(* Logix 5000 Rung export; software revision 16.03 *)

MODULES
   Local : vendor None type None code None
   MCMAOI : vendor None type None code None
END_MODULES

TYPE MCMSTATUS :
STRUCT
   PassCnt : INT;
   Product : INT[2];
   Rev : INT[2];
   OP : INT[2];
   Run : INT[2];
   Prt1Errs : MCMPortErrors;
   Prt2Errs : MCMPortErrors;
   Blk : MCMBlkStat;
   Port1LastErr : INT;
   Port1PreviousErr : INT;
   Port2LastErr : INT;
   Port2PreviousErr : INT;
END_STRUCT
END_TYPE

TYPE MCMCONFIG :
STRUCT
   ModDef : MCMModule;
   Port1 : MCMPort;
   Port2 : MCMPort;
   Port1MasterCmd : MCMCmd[100];
   Port2MasterCmd : MCMCmd[100];
END_STRUCT
END_TYPE

TYPE _CoilArray :
STRUCT
   Boolean : BOOL[416];
END_STRUCT
END_TYPE

TYPE MCMPortErrors :
STRUCT
   CmdReq : INT;
   CmdResp : INT;
   CmdErr : INT;
   Requests : INT;
   Responses : INT;
   ErrSent : INT;
   ErrRec : INT;
END_STRUCT
END_TYPE

TYPE _CmdControl :
STRUCT
   TriggerCmdCntrl : BOOL;
   NumberOfCommands : INT;
   PortNumber : INT;
   CommandIndex : INT[6];
   CmdsAddedToQueue : INT;
   CmdControlBlockID : INT;
   CmdCntrlPending : BOOL;
END_STRUCT
END_TYPE

TYPE _EventCmd :
STRUCT
   EventCmdTrigger : BOOL;
   EventCmdPending : BOOL;
   PortNumber : INT;
   SlaveAddress : INT;
   InternalDBAddress : INT;
   PointCount : INT;
   SwapCode : INT;
   ModbusFunctionCode : INT;
   DeviceDBAddress : INT;
   EventCmdStatusReturned : INT;
   EventBlockID : INT;
END_STRUCT
END_TYPE

TYPE _SlavePollStatus :
STRUCT
   Port1Slave0Read : BOOL;
   Port1Slave128Read : BOOL;
   Port2Slave0Read : BOOL;
   Port2Slave128Read : BOOL;
   P1Slaves : INT[256];
   P2Slaves : INT[256];
END_STRUCT
END_TYPE

TYPE MCMPort :
STRUCT
   Enabled : INT;
   Type : INT;
   FloatFlag : INT;
   FloatStart : INT;
   FloatOffset : INT;
   Protocol : INT;
   Baudrate : INT;
   Parity : INT;
   DataBits : INT;
   StopBits : INT;
   RTSOn : INT;
   RTSOff : INT;
   MinResp : INT;
   UseCTS : INT;
   SlaveID : INT;
   BitInOffset : INT;
   WordInOffset : INT;
   OutOffset : INT;
   HoldOffset : INT;
   CmdCount : INT;
   MinCmdDelay : INT;
   CmdErrPtr : INT;
   RespTO : INT;
   RetryCount : INT;
   ErrorDelayCntr : INT;
   Reserved : INT;
   InterCharacterDelay : INT;
   Fcn99Offset : INT;
END_STRUCT
END_TYPE

TYPE MCMModuleDef :
STRUCT
   CONFIG : MCMCONFIG;
   DATA : MCMDATA;
   STATUS : MCMSTATUS;
   CONTROL : MCMCONTROL;
   _UTIL : _Util;
END_STRUCT
END_TYPE

TYPE MCMCONTROL :
STRUCT
   WarmBoot : BOOL;
   ColdBoot : BOOL;
   BPLastRead : INT;
   BPLastWrite : INT;
   BlockIndex : INT;
   ReadDataSize : DINT;
   MaxReadBlock : DINT;
   WriteDataSize : DINT;
   MaxWriteBlock : DINT;
END_STRUCT
END_TYPE

TYPE MCMModule :
STRUCT
   WriteStartReg : INT;
   WriteRegCnt : INT;
   ReadStartReg : INT;
   ReadRegCnt : INT;
   BPFail : INT;
   ErrStatPtr : INT;
END_STRUCT
END_TYPE

TYPE _Passthru :
STRUCT
   MBOffset : INT;
   MBOffsetBit : INT;
   MBMsgLen : INT;
   MBMsg : SINT[500];
   MBControl1 : CONTROL;
   MBControl2 : CONTROL;
   MBScratch : INT[3];
   MBCoil : _CoilArray;
END_STRUCT
END_TYPE

TYPE MCMDATA :
STRUCT
   ReadData : INT[600];
   WriteData : INT[600];
END_STRUCT
END_TYPE

TYPE MCMBlkStat :
STRUCT
   Read : INT;
   Write : INT;
   Parse : INT;
   Event : INT;
   Cmd : INT;
   Err : INT;
END_STRUCT
END_TYPE

TYPE MCMCmd :
STRUCT
   Enable : INT;
   IntAddress : INT;
   PollInt : INT;
   Count : INT;
   Swap : INT;
   Node : INT;
   Func : INT;
   DevAddress : INT;
END_STRUCT
END_TYPE

TYPE _Util :
STRUCT
   CmdControl : _CmdControl;
   EventCmd : _EventCmd;
   SlavePollStat : _SlavePollStatus;
   Passthru : _Passthru;
END_STRUCT
END_TYPE

ADD_ON_INSTRUCTION PSMCM   (* revision 2.2, vendor ProSoft Technology Inc., ExecutePrescan *)
// Revision note:
// Added viewing capability for the Add_On Instruction
VAR_IN_OUT
   Local_C : SINT[400]; {required}
   Local_Input : INT[250]; {required}
   Local_Output : INT[248]; {required}
   MCM : MCMModuleDef; {required}
END_VAR
VAR
   MJFAULTS : DINT[12];
END_VAR

ROUTINE Logic   (* ladder *)
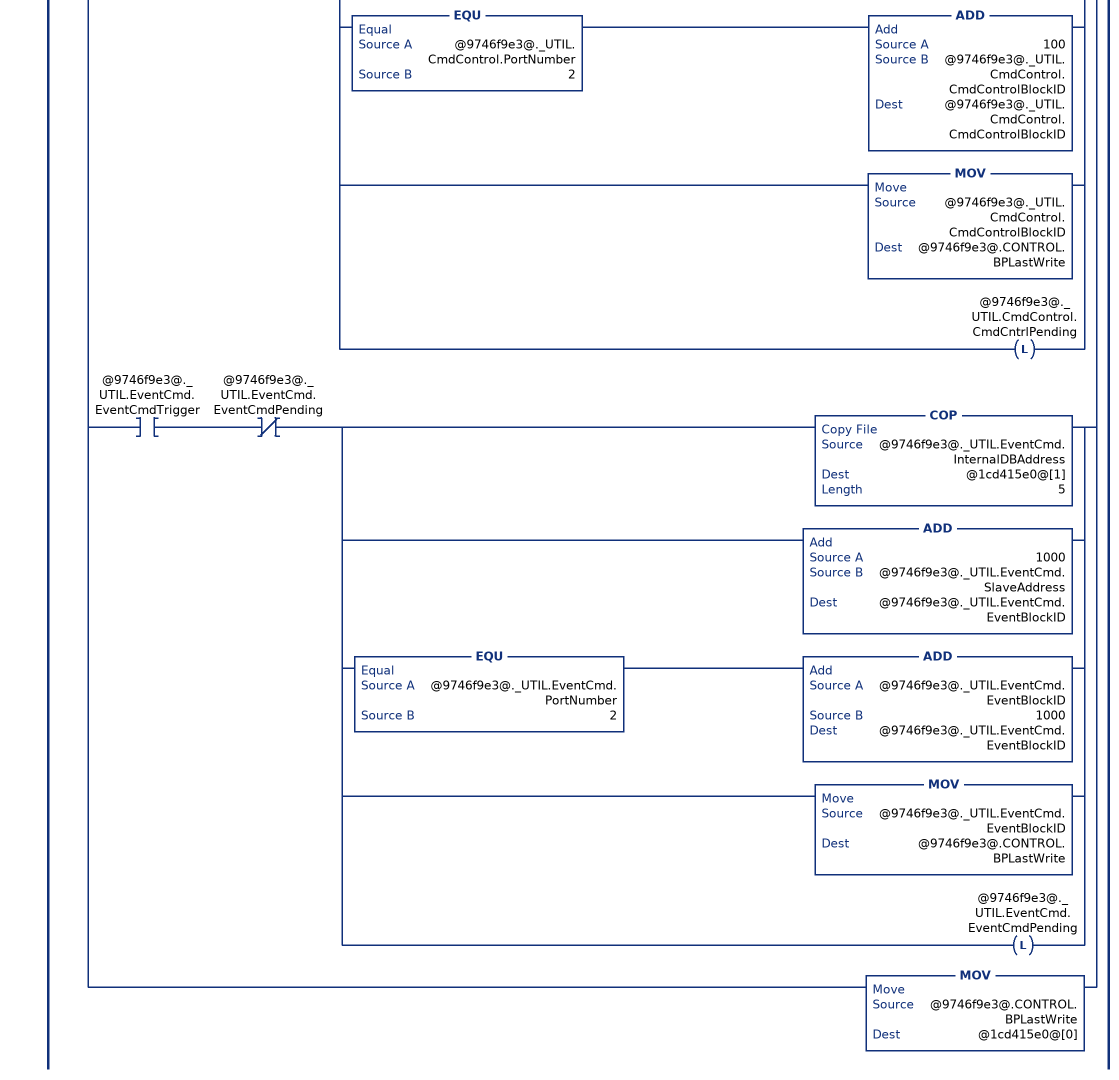
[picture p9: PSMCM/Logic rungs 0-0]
   0: NEQ(@5153acc1@[249],@9746f9e3@.CONTROL.BPLastRead)[MOV(@5153acc1@[249],@9746f9e3@.CONTROL.BPLastRead) ,[EQU(-1,@9746f9e3@.CONTROL.BPLastRead) ,EQU(0,@9746f9e3@.CONTROL.BPLastRead) ] [COP(@5153acc1@[202],@9746f9e3@.STATUS.PassCnt,1) ,COP(@5153acc1@[203],@9746f9e3@.STATUS.Product[0],8) ,COP(@5153acc1@[211],@9746f9e3@.STATUS.Prt1Errs.CmdReq,7) ,COP(@5153acc1@[218],@9746f9e3@.STATUS.Prt2Errs.CmdReq,7) ,COP(@5153acc1@[225],@9746f9e3@.STATUS.Blk.Read,6) ,COP(@5153acc1@[231],@9746f9e3@.STATUS.Port1LastErr,4) ] ,LIM(1,@9746f9e3@.CONTROL.BPLastRead,@9746f9e3@.CONTROL.MaxReadBlock) [CPT(@9746f9e3@.CONTROL.BlockIndex,(@9746f9e3@.CONTROL.BPLastRead-1)*200) ,COP(@5153acc1@[2],@9746f9e3@.DATA.ReadData[@9746f9e3@.CONTROL.BlockIndex],200) ,COP(@5153acc1@[202],@9746f9e3@.STATUS.PassCnt,1) ,COP(@5153acc1@[203],@9746f9e3@.STATUS.Product[0],8) ,COP(@5153acc1@[211],@9746f9e3@.STATUS.Prt1Errs.CmdReq,7) ,COP(@5153acc1@[218],@9746f9e3@.STATUS.Prt2Errs.CmdReq,7) ,COP(@5153acc1@[225],@9746f9e3@.STATUS.Blk.Read,6) ,COP(@5153acc1@[231],@9746f9e3@.STATUS.Port1LastErr,4) ] ,EQU(9996,@9746f9e3@.CONTROL.BPLastRead) [MOV(@5153acc1@[2],@9746f9e3@._UTIL.Passthru.MBMsgLen) ,COP(@5153acc1@[4],@9746f9e3@._UTIL.Passthru.MBMsg[0],@9746f9e3@._UTIL.Passthru.MBMsgLen) ] ,LIM(9956,@9746f9e3@.CONTROL.BPLastRead,9957) [MOV(@5153acc1@[3],@9746f9e3@._UTIL.Passthru.MBOffset) ,COP(@5153acc1@[4],@9746f9e3@.DATA.WriteData[@9746f9e3@._UTIL.Passthru.MBOffset],@5153acc1@[2]) ] ,EQU(9958,@9746f9e3@.CONTROL.BPLastRead) LES(@5153acc1@[3],416) [MOV(@5153acc1@[3],@9746f9e3@._UTIL.Passthru.MBOffsetBit) ,MOV(@5153acc1@[4],@9746f9e3@._UTIL.Passthru.MBScratch[2]) ,COP(@9746f9e3@.DATA.WriteData[0],@9746f9e3@._UTIL.Passthru.MBCoil,1) ,NEQ(@9746f9e3@._UTIL.Passthru.MBScratch[2],0) OTL(@9746f9e3@._UTIL.Passthru.MBCoil.Boolean[@9746f9e3@._UTIL.Passthru.MBOffsetBit]) ,EQU(@9746f9e3@._UTIL.Passthru.MBScratch[2],0) OTU(@9746f9e3@._UTIL.Passthru.MBCoil.Boolean[@9746f9e3@._UTIL.Passthru.MBOffsetBit]) ,COP(@9746f9e3@._UTIL.Passthru.MBCoil,@9746f9e3@.DATA.WriteData[0],26) ] ,EQU(9959,@9746f9e3@.CONTROL.BPLastRead) [MOV(@5153acc1@[3],@9746f9e3@._UTIL.Passthru.MBOffset) ,MOV(@5153acc1@[2],@9746f9e3@._UTIL.Passthru.MBControl1.LEN) ,MOV(@5153acc1@[2],@9746f9e3@._UTIL.Passthru.MBControl2.LEN) ,FAL(@9746f9e3@._UTIL.Passthru.MBControl1,?,?,ALL,@9746f9e3@.DATA.WriteData[@9746f9e3@._UTIL.Passthru.MBOffset+@9746f9e3@._UTIL.Passthru.MBControl1.POS],@9746f9e3@.DATA.WriteData[@9746f9e3@._UTIL.Passthru.MBOffset+@9746f9e3@._UTIL.Passthru.MBControl1.POS] AND(NOT @5153acc1@[54+@9746f9e3@._UTIL.Passthru.MBControl1.POS])) ,FAL(@9746f9e3@._UTIL.Passthru.MBControl2,?,?,ALL,@9746f9e3@.DATA.WriteData[@9746f9e3@._UTIL.Passthru.MBOffset+@9746f9e3@._UTIL.Passthru.MBControl2.POS],@9746f9e3@.DATA.WriteData[@9746f9e3@._UTIL.Passthru.MBOffset+@9746f9e3@._UTIL.Passthru.MBControl2.POS] OR(@5153acc1@[54+@9746f9e3@._UTIL.Passthru.MBControl2.POS] AND @5153acc1@[4+@9746f9e3@._UTIL.Passthru.MBControl2.POS])) ,RES(@9746f9e3@._UTIL.Passthru.MBControl1) ,RES(@9746f9e3@._UTIL.Passthru.MBControl2) ] ,LIM(3002,@9746f9e3@.CONTROL.BPLastRead,3003) [CPT(@9746f9e3@.CONTROL.BlockIndex,(@9746f9e3@.CONTROL.BPLastRead-3002)*128) ,COP(@5153acc1@[2],@9746f9e3@._UTIL.SlavePollStat.P1Slaves[@9746f9e3@.CONTROL.BlockIndex],128) ] ,LIM(3102,@9746f9e3@.CONTROL.BPLastRead,3103) [CPT(@9746f9e3@.CONTROL.BlockIndex,(@9746f9e3@.CONTROL.BPLastRead-3102)*128) ,COP(@5153acc1@[2],@9746f9e3@._UTIL.SlavePollStat.P2Slaves[@9746f9e3@.CONTROL.BlockIndex],128) ] ,[LIM(5001,@9746f9e3@.CONTROL.BPLastRead,5006) ,LIM(5101,@9746f9e3@.CONTROL.BPLastRead,5106) ] [MOV(@5153acc1@[2],@9746f9e3@._UTIL.CmdControl.CmdsAddedToQueue) ,OTU(@9746f9e3@._UTIL.CmdControl.CmdCntrlPending) ,OTU(@9746f9e3@._UTIL.CmdControl.TriggerCmdCntrl) ] ,[LIM(1000,@9746f9e3@.CONTROL.BPLastRead,1255) ,LIM(2000,@9746f9e3@.CONTROL.BPLastRead,2255) ] [MOV(@5153acc1@[2],@9746f9e3@._UTIL.EventCmd.EventCmdStatusReturned) ,OTU(@9746f9e3@._UTIL.EventCmd.EventCmdPending) ,OTU(@9746f9e3@._UTIL.EventCmd.EventCmdTrigger) ] ,EQU(-9000,@9746f9e3@.CONTROL.BPLastRead) [COP(@5153acc1@[2],@9746f9e3@.CONFIG.ModDef.WriteStartReg,6) ,COP(@5153acc1@[8],@9746f9e3@.CONFIG.Port1.Enabled,25) ,COP(@5153acc1@[33],@9746f9e3@.CONFIG.Port2.Enabled,25) ,COP(@5153acc1@[58],@9746f9e3@.CONFIG.Port1.Reserved,3) ,COP(@5153acc1@[61],@9746f9e3@.CONFIG.Port2.Reserved,3) ,MOV(@9746f9e3@.CONTROL.BPLastRead,@1cd415e0@[0]) ] ,LIM(-6003,@9746f9e3@.CONTROL.BPLastRead,-6000) [CPT(@9746f9e3@.CONTROL.BPLastWrite,(-@9746f9e3@.CONTROL.BPLastRead-6000)*25) ,COP(@5153acc1@[2],@9746f9e3@.CONFIG.Port1MasterCmd[@9746f9e3@.CONTROL.BPLastWrite].Enable,200) ,MOV(@9746f9e3@.CONTROL.BPLastRead,@1cd415e0@[0]) ] ,LIM(-6103,@9746f9e3@.CONTROL.BPLastRead,-6100) [CPT(@9746f9e3@.CONTROL.BPLastWrite,(-@9746f9e3@.CONTROL.BPLastRead-6100)*25) ,COP(@5153acc1@[2],@9746f9e3@.CONFIG.Port2MasterCmd[@9746f9e3@.CONTROL.BPLastWrite].Enable,200) ,MOV(@9746f9e3@.CONTROL.BPLastRead,@1cd415e0@[0]) ] ,MOV(@5153acc1@[1],@9746f9e3@.CONTROL.BPLastWrite) ,XIC(@9746f9e3@.CONTROL.WarmBoot) [MOV(9998,@9746f9e3@.CONTROL.BPLastWrite) ,OTU(@9746f9e3@.CONTROL.WarmBoot) ] ,XIC(@9746f9e3@.CONTROL.ColdBoot) [MOV(9999,@9746f9e3@.CONTROL.BPLastWrite) ,OTU(@9746f9e3@.CONTROL.ColdBoot) ] ,LIM(1,@9746f9e3@.CONTROL.BPLastWrite,@9746f9e3@.CONTROL.MaxWriteBlock) [CPT(@9746f9e3@.CONTROL.BlockIndex,(@9746f9e3@.CONTROL.BPLastWrite-1)*200) ,COP(@9746f9e3@.DATA.WriteData[@9746f9e3@.CONTROL.BlockIndex],@1cd415e0@[1],200) ] ,EQU(9000,@9746f9e3@.CONTROL.BPLastWrite) [COP(@9746f9e3@.CONFIG.ModDef.WriteStartReg,@1cd415e0@[1],6) ,COP(@9746f9e3@.CONFIG.Port1.Enabled,@1cd415e0@[7],25) ,COP(@9746f9e3@.CONFIG.Port2.Enabled,@1cd415e0@[32],25) ,COP(@9746f9e3@.CONFIG.Port1.Reserved,@1cd415e0@[57],3) ,COP(@9746f9e3@.CONFIG.Port2.Reserved,@1cd415e0@[60],3) ] ,LIM(6000,@9746f9e3@.CONTROL.BPLastWrite,6003) [CPT(@9746f9e3@.CONTROL.BlockIndex,(@9746f9e3@.CONTROL.BPLastWrite-6000)*25) ,COP(@9746f9e3@.CONFIG.Port1MasterCmd[@9746f9e3@.CONTROL.BlockIndex].Enable,@1cd415e0@[1],200) ] ,LIM(6100,@9746f9e3@.CONTROL.BPLastWrite,6103) [CPT(@9746f9e3@.CONTROL.BlockIndex,(@9746f9e3@.CONTROL.BPLastWrite-6100)*25) ,COP(@9746f9e3@.CONFIG.Port2MasterCmd[@9746f9e3@.CONTROL.BlockIndex].Enable,@1cd415e0@[1],200) ] ,XIC(@9746f9e3@._UTIL.SlavePollStat.Port1Slave0Read) [MOV(3002,@9746f9e3@.CONTROL.BPLastWrite) ,OTU(@9746f9e3@._UTIL.SlavePollStat.Port1Slave0Read) ] ,XIC(@9746f9e3@._UTIL.SlavePollStat.Port1Slave128Read) [MOV(3003,@9746f9e3@.CONTROL.BPLastWrite) ,OTU(@9746f9e3@._UTIL.SlavePollStat.Port1Slave128Read) ] ,XIC(@9746f9e3@._UTIL.SlavePollStat.Port2Slave0Read) [MOV(3102,@9746f9e3@.CONTROL.BPLastWrite) ,OTU(@9746f9e3@._UTIL.SlavePollStat.Port2Slave0Read) ] ,XIC(@9746f9e3@._UTIL.SlavePollStat.Port2Slave128Read) [MOV(3103,@9746f9e3@.CONTROL.BPLastWrite) ,OTU(@9746f9e3@._UTIL.SlavePollStat.Port2Slave128Read) ] ,XIC(@9746f9e3@._UTIL.CmdControl.TriggerCmdCntrl) XIO(@9746f9e3@._UTIL.CmdControl.CmdCntrlPending) [COP(@9746f9e3@._UTIL.CmdControl.CommandIndex[0],@1cd415e0@[1],6) ,ADD(5000,@9746f9e3@._UTIL.CmdControl.NumberOfCommands,@9746f9e3@._UTIL.CmdControl.CmdControlBlockID) ,EQU(@9746f9e3@._UTIL.CmdControl.PortNumber,2) ADD(100,@9746f9e3@._UTIL.CmdControl.CmdControlBlockID,@9746f9e3@._UTIL.CmdControl.CmdControlBlockID) ,MOV(@9746f9e3@._UTIL.CmdControl.CmdControlBlockID,@9746f9e3@.CONTROL.BPLastWrite) ,OTL(@9746f9e3@._UTIL.CmdControl.CmdCntrlPending) ] ,XIC(@9746f9e3@._UTIL.EventCmd.EventCmdTrigger) XIO(@9746f9e3@._UTIL.EventCmd.EventCmdPending) [COP(@9746f9e3@._UTIL.EventCmd.InternalDBAddress,@1cd415e0@[1],5) ,ADD(1000,@9746f9e3@._UTIL.EventCmd.SlaveAddress,@9746f9e3@._UTIL.EventCmd.EventBlockID) ,EQU(@9746f9e3@._UTIL.EventCmd.PortNumber,2) ADD(@9746f9e3@._UTIL.EventCmd.EventBlockID,1000,@9746f9e3@._UTIL.EventCmd.EventBlockID) ,MOV(@9746f9e3@._UTIL.EventCmd.EventBlockID,@9746f9e3@.CONTROL.BPLastWrite) ,OTL(@9746f9e3@._UTIL.EventCmd.EventCmdPending) ] ,MOV(@9746f9e3@.CONTROL.BPLastWrite,@1cd415e0@[0]) ];
END_ROUTINE

ROUTINE Prescan   (* ladder *)
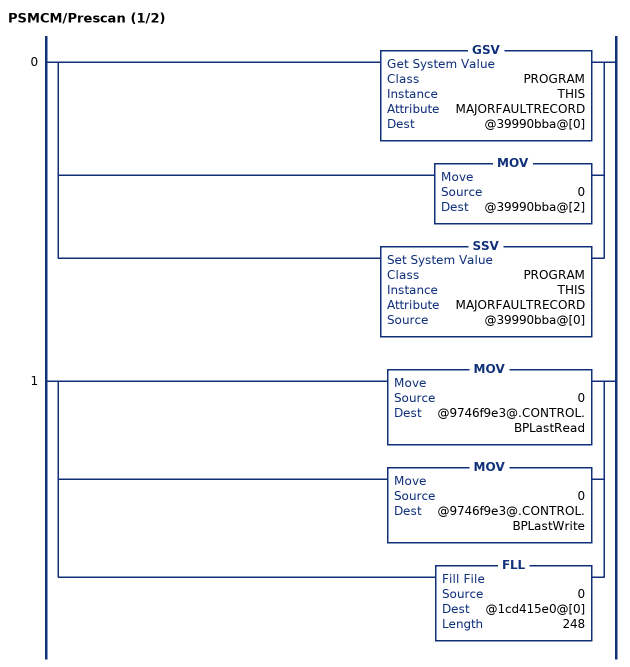
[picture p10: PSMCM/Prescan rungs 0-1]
   0: [GSV(PROGRAM,THIS,MAJORFAULTRECORD,@39990bba@[0]) ,MOV(0,@39990bba@[2]) ,SSV(PROGRAM,THIS,MAJORFAULTRECORD,@39990bba@[0]) ];
   1: [MOV(0,@9746f9e3@.CONTROL.BPLastRead) ,MOV(0,@9746f9e3@.CONTROL.BPLastWrite) ,FLL(0,@1cd415e0@[0],248) ];
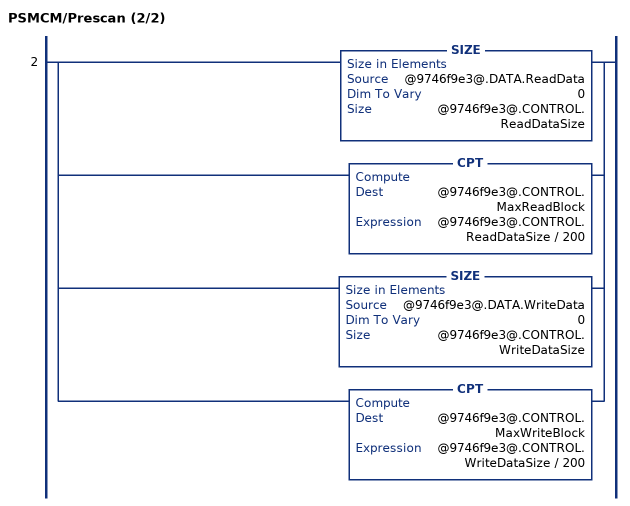
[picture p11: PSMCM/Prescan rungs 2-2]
   2: [SIZE(@9746f9e3@.DATA.ReadData,0,@9746f9e3@.CONTROL.ReadDataSize) ,CPT(@9746f9e3@.CONTROL.MaxReadBlock,@9746f9e3@.CONTROL.ReadDataSize / 200) ,SIZE(@9746f9e3@.DATA.WriteData,0,@9746f9e3@.CONTROL.WriteDataSize) ,CPT(@9746f9e3@.CONTROL.MaxWriteBlock,@9746f9e3@.CONTROL.WriteDataSize / 200) ];
END_ROUTINE
END_ADD_ON_INSTRUCTION

VAR_GLOBAL   (* controller tags *)
   Local:3:O : AB:1756_MODULE_INT_496Bytes:O:0;
   Local:3:I : AB:1756_MODULE_INT_500Bytes:I:0;
   MCM : MCMModuleDef;
   Local:3:C : AB:1756_MODULE:C:0;
   PSMCM : PSMCM;
END_VAR

PROGRAM MainProgram

ROUTINE MainRoutine   (* ladder *)
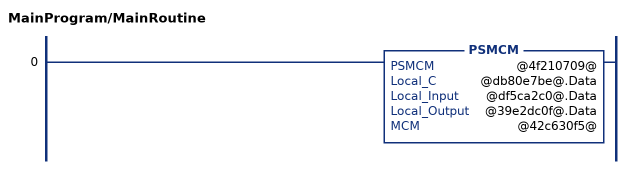
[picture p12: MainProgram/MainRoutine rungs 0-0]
   0: PSMCM(@4f210709@,@db80e7be@.Data,@df5ca2c0@.Data,@39e2dc0f@.Data,@42c630f5@);
END_ROUTINE
END_PROGRAM
